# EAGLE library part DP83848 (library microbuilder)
DP83848 (40-LLP) - Single Port 10/100 Ethernet Transceiver Digikey: DP83848JSQCT-ND
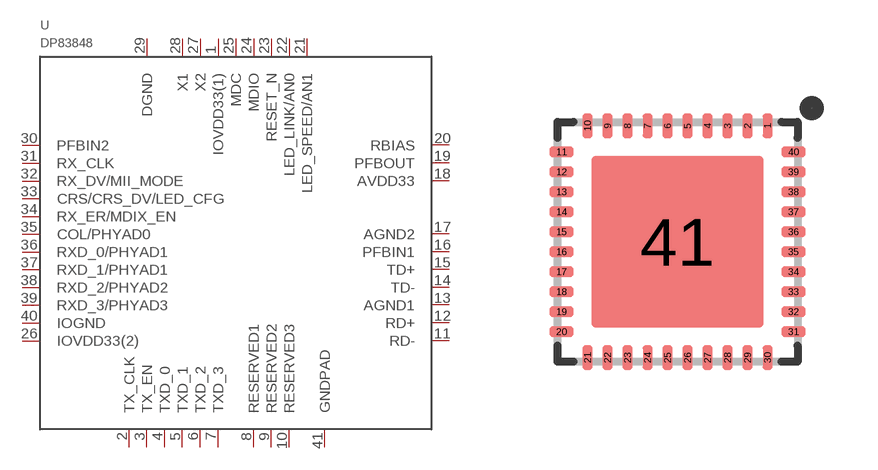
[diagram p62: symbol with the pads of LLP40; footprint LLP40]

Designator prefix U

## DP83848  [LLP40]
1  IOVDD33(1)
2  TX_CLK
3  TX_EN
4  TXD_0
5  TXD_1
6  TXD_2
7  TXD_3
8  RESERVED1
9  RESERVED2
10  RESERVED3
11  RD-
12  RD+
13  AGND1
14  TD-
15  TD+
16  PFBIN1
17  AGND2
18  AVDD33
19  PFBOUT
20  RBIAS
21  LED_SPEED/AN1
22  LED_LINK/AN0
23  RESET_N
24  MDIO
25  MDC
26  IOVDD33(2)
27  X2
28  X1
29  DGND
30  PFBIN2
31  RX_CLK
32  RX_DV/MII_MODE
33  CRS/CRS_DV/LED_CFG
34  RX_ER/MDIX_EN
35  COL/PHYAD0
36  RXD_0/PHYAD1
37  RXD_1/PHYAD1
38  RXD_2/PHYAD2
39  RXD_3/PHYAD3
40  IOGND
41  GNDPAD

## Footprint LLP40 (pad centres in mm)
40-LLP Package Source: http://cache.national.com/ds/DP/DP83848J.pdf
smd 0.25 x 0.6: 1 2.25,2.9; 2 1.75,2.9; 3 1.25,2.9; 4 0.75,2.9; 5 0.25,2.9; 6 -0.25,2.9; 7 -0.75,2.9; 8 -1.25,2.9; 9 -1.75,2.9; 10 -2.25,2.9; 21 -2.25,-2.9; 22 -1.75,-2.9; 23 -1.25,-2.9; 24 -0.75,-2.9; 25 -0.25,-2.9; 26 0.25,-2.9; 27 0.75,-2.9; 28 1.25,-2.9; 29 1.75,-2.9; 30 2.25,-2.9
smd 0.6 x 0.25: 11 -2.9,2.25; 12 -2.9,1.75; 13 -2.9,1.25; 14 -2.9,0.75; 15 -2.9,0.25; 16 -2.9,-0.25; 17 -2.9,-0.75; 18 -2.9,-1.25; 19 -2.9,-1.75; 20 -2.9,-2.25; 31 2.9,-2.25; 32 2.9,-1.75; 33 2.9,-1.25; 34 2.9,-0.75; 35 2.9,-0.25; 36 2.9,0.25; 37 2.9,0.75; 38 2.9,1.25; 39 2.9,1.75; 40 2.9,2.25
smd 4.3 x 4.3: 41 0,0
